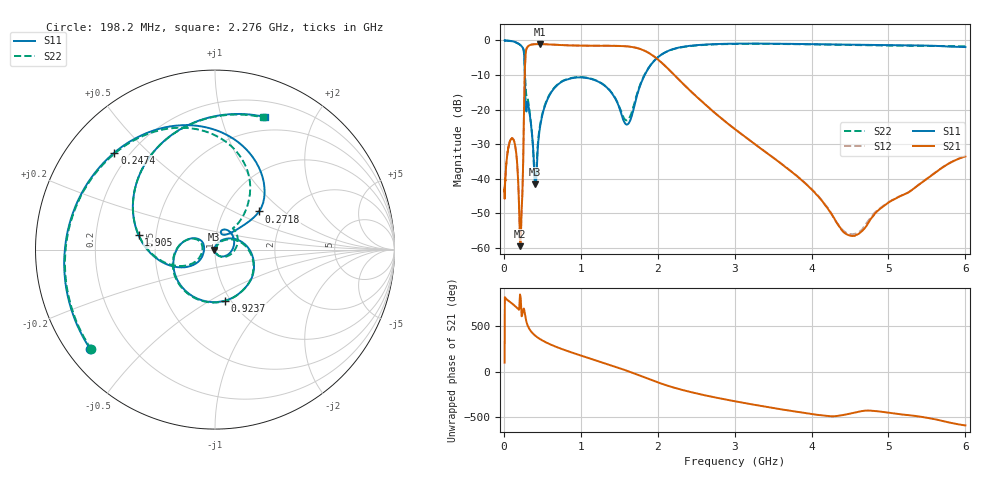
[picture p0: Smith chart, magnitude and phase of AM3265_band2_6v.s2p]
!Agilent Technologies,E8364B,MY43040894,A.07.50.67
!Agilent E8364B: A.07.50.67
!Date: Friday, May 09, 2025 07:25:17
!Correction: S11(Full 2 Port(1,2))
!S21(Full 2 Port(1,2))
!S12(Full 2 Port(1,2))
!S22(Full 2 Port(1,2))
!S2P File: Measurements: S11, S21, S12, S22:Log Frequency Sweep
# Hz S  dB  R 50
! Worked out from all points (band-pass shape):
!   3201 points, 10 MHz to 6 GHz, reference 50 ohm
!   highest |S21| = -1.06 dB at 464.4 MHz (marker M1); lowest = -59.5 dB at 214.7 MHz (marker M2)
!   |S21| within 3 dB of the highest: 283.1 MHz to 1.916 GHz (1.633 GHz wide, 149 % of centre)
!   lowest |S11| = -41.6 dB at 409.4 MHz (marker M3), VSWR 1.02, Z = 49.2 - j0.0526 ohm
!   |S11| at or under -10 dB: 272 MHz to 1.831 GHz (1.559 GHz wide, 148 % of centre)
!   |S22| runs from -40.3 to 0.0 dB; largest |S21 - S12| = 0.014
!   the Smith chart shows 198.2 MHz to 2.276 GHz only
!   S11 on the Smith chart (normalised r, x): 198.2 MHz: 0.07, -0.35; 247.4 MHz: 0.14, +0.40; 271.8 MHz: 1.46, +0.69; 923.7 MHz: 0.94, -0.59; 1.905 GHz: 0.40, +0.08; 2.276 GHz: 0.35, +1.39
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1e7  -0.01 -5.7  -42.93 99.9  -41.69 92.1  -0.07 -5.6
2.908064e7  -0.04 -16.2  -36.57 75.7  -36.40 74.8  -0.04 -16.3
8.439949e7  -0.12 -48.4  -28.85 40.9  -28.89 40.8  -0.16 -48.7
1.981752e8  -1.03 -141.6  -48.34 -40.4  -48.70 -38.3  -1.06 -141.2
2.146724e8  -1.31 -162.9  -59.49 109.2  -58.04 -88.5  -1.34 -162.0
2.44949e8  -2.08 142.2  -41.36 -71.3  -41.47 -73.1  -2.07 145.8
2.474096e8  -2.17 136.0  -39.26 -60.6  -39.29 -62.9  -2.16 140.1
2.717819e8  -9.77 40.9  -9.86 -74.8  -9.83 -74.8  -7.52 62.4
3.027624e8  -18.01 62.8  -2.03 160.7  -1.99 160.6  -16.31 43.3
4.094453e8  -41.60 -176.3  -1.08 33.5  -1.04 33.5  -40.30 3.8
4.643984e8  -25.98 61.3  -1.06 0.3  -1.02 0.3  -25.39 53.6
7.123273e8  -12.58 -22.4  -1.30 -98.5  -1.26 -98.5  -12.46 -25.8
9.237235e8  -10.75 -78.8  -1.47 -161.5  -1.44 -161.5  -10.66 -81.5
1.339745e9  -13.62 177.6  -1.54 84.9  -1.51 84.8  -13.56 177.4
1.904673e9  -7.26 169.3  -3.89 -86.5  -3.87 -86.5  -7.18 168.3
2.067357e9  -3.81 121.7  -6.76 -136.0  -6.73 -136.0  -3.83 121.9
2.275557e9  -2.05 69.2  -11.33 170.4  -11.31 170.4  -2.12 70.0
3.202913e9  -0.90 -91.4  -29.01 6.0  -28.98 5.9  -0.97 -91.5
3.818953e9  -1.01 -178.1  -39.38 -80.8  -39.32 -80.4  -1.08 -179.7
4.499191e9  -1.22 90.8  -56.44 -98.4  -56.05 -98.8  -1.30 89.3
5.195685e9  -1.41 -0.1  -44.61 -110.1  -44.61 -109.9  -1.52 -0.0
6e9  -1.91 -96.9  -33.55 131.8  -33.54 132.0  -1.68 -96.5
